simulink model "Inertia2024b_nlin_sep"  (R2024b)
settings: Solver=ode1  StartTime=0.0  StopTime=30  FixedStep=Tstep  EnableMultiTasking=on
model workspace (MAT data in the model file):
  op_snapshot1 : opcond.OperatingPoint (value not decoded)
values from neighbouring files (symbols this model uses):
  T_dis = 2.5    [onebus_nonlinsub.m]
  Ts = Tstep    (= 1e-05)    [onebus_nonlinsub.m]    (also in DemoMTI_Boolean_Index_MTI.m = 1; DemoMTI_EKF.m = 0.02; DemoMTI_MHE_VanDePol.m = 0.01)
  Tstep = 1e-5    (= 1e-05)    [DemoMTI_greyestGFM.m]    (also in onebus_nonlinsub.m)
  Vn = 380    [simulink_parameters_one_bus.m]    (also in nine_bus_parameters.m = 310.*ones(num_inv,1))
  Vtri = Vdc1./3    [simulink_parameters_one_bus.m]    (also in nine_bus_parameters.m = Vdc./2)
  wn = ones(num_inv,1).*w01    [nine_bus_parameters.m]    (also in computeModeFrequencyDampingTable.m = abs(lambda))
undefined symbols (not defined in the file or in its folder): D1_g1, Dsg, Dxd, Dxq, Efdmax_g1, Efdmin_g1, Ibg, K_int_pll, K_prop_pll, KA_g1, kpss_g1, L_1_2, M1_g1, Msg, nom, op, R_1_2, ra_g1, Rsg, T1_g1, T2_g1, T3_g1, T4_g1, TA_g1, Td, Td0p_g1, Tq0p_g1, Tv, Tw_g1, Vbg, xdp_g1, xqp_g1
libraries: spsThreePhaseVIMeasurementLib x5, spsGroundLib x4, slpidlib x4, spsControlledVoltageSourceLib x3, spsControlledCurrentSourceLib x3, spsSeriesRLCBranchLib x3, spsThreePhaseSeriesRLCBranchLib x2, spsThreePhaseSeriesRLCLoadLib x2, spsThreePhaseTransformerTwoWindingsLib x1, spsThreePhaseDynamicLoadLib x1, spsSampleandHoldLib x1, sps_lib x1
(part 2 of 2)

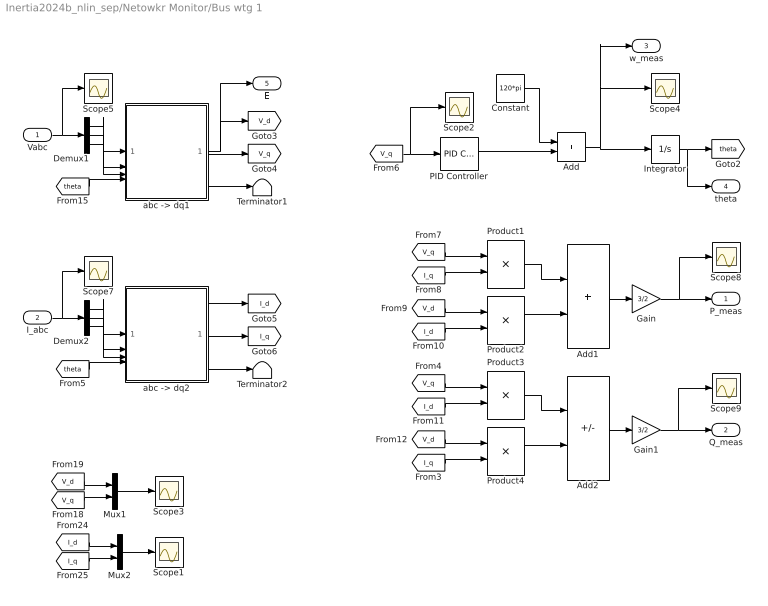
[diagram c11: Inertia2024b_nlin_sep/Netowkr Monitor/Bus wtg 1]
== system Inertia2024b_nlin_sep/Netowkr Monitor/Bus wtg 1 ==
  Vabc : Inport
  I_abc : Inport  Port=2
  Add : Sum
  Add1 : Sum
  Add2 : Sum  Inputs=+-
  Constant : Constant  Value=120*pi
  Demux1 : Demux  Outputs=3
  Demux2 : Demux  Outputs=3
  Gain : Gain  Gain=3/2
  Gain1 : Gain  Gain=3/2
  Integrator : Integrator  IgnoreLimit=on
  Mux1 : Mux  Inputs=2
  Mux2 : Mux  Inputs=2
  PID Controller : slpidlib/PID Controller  Controller=PI  Form=Parallel  TimeDomain=Continuous-time  UseExternalTs=off  SampleTime=-1  IntegratorMethod=Forward Euler  FilterMethod=Forward Euler  ControllerParametersSource=internal  P=K_prop_pll  I=K_int_pll  UseKiTs=off  D=0  UseExternalDerivativeSource=off  N=100  UseFilter=on  TunerSelectOption=Transfer Function Based (PID Tuner App)  InitialConditionSource=internal  InitialConditionForIntegrator=0  InitialConditionForFilter=0  DifferentiatorICPrevScaledInput=0  ExternalReset=none  IgnoreLimit=on  TrackingMode=off  Kt=1  LimitOutput=off  SatLimitsSource=internal  UpperSaturationLimit=inf  LowerSaturationLimit=-inf  LinearizeAsGain=on  AntiWindupMode=none  Kb=1  LimitIntegrator=off  UpperIntegratorSaturationLimit=inf  LowerIntegratorSaturationLimit=-inf  POutMin=[]  POutMax=[]  IOutMin=[]  IOutMax=[]  DOutMin=[]  DOutMax=[]  NOutMin=[]  NOutMax=[]  SumOutMin=[]  SumOutMax=[]  SaturationOutMin=[]  SaturationOutMax=[]  PParamMin=[]  PParamMax=[]  IParamMin=[]  IParamMax=[]  DParamMin=[]  DParamMax=[]  NParamMin=[]  NParamMax=[]  KbParamMin=[]  KbParamMax=[]  KtParamMin=[]  KtParamMax=[]  KbOutMin=[]  KbOutMax=[]  KtOutMin=[]  KtOutMax=[]  IntegratorOutMin=[]  IntegratorOutMax=[]  FilterOutMin=[]  FilterOutMax=[]  SumI1OutMin=[]  SumI1OutMax=[]  SumI2OutMin=[]  SumI2OutMax=[]  SumI3OutMin=[]  SumI3OutMax=[]  SumI4OutMin=[]  SumI4OutMax=[]  SumDOutMin=[]  SumDOutMax=[]  DifferentiatorOutMin=[]  DifferentiatorOutMax=[]  FilterDiffOutCoefMin=[]  FilterDiffOutCoefMax=[]  ReciprocalOutMin=[]  ReciprocalOutMax=[]  SumDenOutMin=[]  SumDenOutMax=[]  SumNumOutMin=[]  SumNumOutMax=[]  DivideOutMin=[]  DivideOutMax=[]  UdiffTsProdOutMin=[]  UdiffTsProdOutMax=[]  NTsProdOutMin=[]  NTsProdOutMax=[]  UintegralTsProdOutMin=[]  UintegralTsProdOutMax=[]  UngainTsProdOutMin=[]  UngainTsProdOutMax=[]  ClampingZeroOutDataTypeStr=Inherit: Inherit via back propagation  ClampingZeroOutMin=[]  ClampingZeroOutMax=[]  FilterDenConstantOutDataTypeStr=Inherit: Inherit via back propagation  FilterDenConstantOutMin=[]  FilterDenConstantOutMax=[]  PCopyOutDataTypeStr=Inherit: Inherit via back propagation  PCopyOutMin=[]  PCopyOutMax=[]  NCopyOutDataTypeStr=Inherit: Inherit via back propagation  NCopyOutMin=[]  NCopyOutMax=[]  IntegratorContinuousStateAttributes=''  IntegratorStateMustResolveToSignalObject=off  IntegratorRTWStateStorageClass=Auto  FilterContinuousStateAttributes=''  FilterStateMustResolveToSignalObject=off  FilterRTWStateStorageClass=Auto  ParallelPVariant=InternalParameters  IdealPVariant=Disabled  IVariant=InternalParameters  DVariant=Disabled  IntegratorVariant=Continuous  SatVariant=Disabled  AWVariant=Passthrough  PCopyVariant=Disabled  TRVariant=Disabled  FdbkBlocksVariant=Forward  IdealPFdbkVariant=Disabled  SatFdbkVariant=Disabled  DerivativeFilterVariant=Disabled  NVariant=Disabled  NCopyVariant=Disabled_SignalSpec  FilterICVariant=Disabled  IntegratorICVariant=InternalICs  ExternalResetVariant=Disabled  TRSumVariant=Passthrough  SumFdbkVariant=Disabled  SumVariant=Sum_PI  TsampFilterVariant=InternalTs  TsampNgainVariant=Passthrough  TsampIntegralVariant=Disabled_SignalSpec  ExternalSaturationOutDataTypeStr=Inherit: Same as second input  DerivativeSourceVariant=Disabled  PreIntVariant=InternalPreInt
  Product{1..4} (4 alike) : Product
  Scope{1..5,7..9} (8 alike) : Scope
  Terminator1 : Terminator
  Terminator2 : Terminator
  "abc -> dq1" : Subsystem
  "abc -> dq2" : Subsystem
  P_meas : Outport  VectorParamsAs1DForOutWhenUnconnected=off
  Q_meas : Outport  Port=2  VectorParamsAs1DForOutWhenUnconnected=off
  w_meas : Outport  Port=3  VectorParamsAs1DForOutWhenUnconnected=off
  theta : Outport  Port=4  VectorParamsAs1DForOutWhenUnconnected=off
  E : Outport  Port=5  VectorParamsAs1DForOutWhenUnconnected=off
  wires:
  Add/1 -> Integrator/1, w_meas/1, Scope4/1
  [V_q] -> Scope2/1, PID Controller/1
  PID Controller/1 -> Add/2
  Constant/1 -> Add/1
  Demux1/2 -> "abc -> dq1"/2(b)
  Demux1/3 -> "abc -> dq1"/3(c)
  [theta] -> "abc -> dq1"/4(Theta)
  Vabc/1 -> Scope5/1, Demux1/1
  Demux1/1 -> "abc -> dq1"/1(a)
  "abc -> dq1"/3(0) -> Terminator1/1
  "abc -> dq1"/2(q) -> [V_q]
  Integrator/1 -> theta/1, [theta]
  Demux2/2 -> "abc -> dq2"/2(b)
  Demux2/3 -> "abc -> dq2"/3(c)
  [theta] -> "abc -> dq2"/4(Theta)
  I_abc/1 -> Scope7/1, Demux2/1
  Demux2/1 -> "abc -> dq2"/1(a)
  "abc -> dq2"/3(0) -> Terminator2/1
  "abc -> dq2"/2(q) -> [I_q]
  "abc -> dq2"/1(d) -> [I_d]
  [V_q] -> Product1/1
  [I_q] -> Product1/2
  Product1/1 -> Add1/1
  [V_d] -> Product2/1
  [I_d] -> Product2/2
  Product2/1 -> Add1/2
  Add1/1 -> Gain/1
  Gain/1 -> Scope8/1, P_meas/1
  [V_q] -> Product3/1
  [I_d] -> Product3/2
  Product3/1 -> Add2/1
  [V_d] -> Product4/1
  [I_q] -> Product4/2
  Product4/1 -> Add2/2
  Add2/1 -> Gain1/1
  Gain1/1 -> Scope9/1, Q_meas/1
  [V_d] -> Mux1/1
  [I_d] -> Mux2/1
  [I_q] -> Mux2/2
  [V_q] -> Mux1/2
  Mux1/1 -> Scope3/1
  Mux2/1 -> Scope1/1
  "abc -> dq1"/1(d) -> E/1, [V_d]

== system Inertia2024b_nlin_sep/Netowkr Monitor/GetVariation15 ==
  In1 : Inport
  Minus : Sum  Inputs=|+-
  Sample and Hold2 : spsSampleandHoldLib/Sample and Hold  ic=0  Ts=Ts
  Scope17 : Scope
  Out1 : Outport  VectorParamsAs1DForOutWhenUnconnected=off
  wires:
  Sample and Hold2/1 -> Scope17/1, Minus/2
  [op_hold] -> Sample and Hold2/2
  In1/1 -> Sample and Hold2/1, Minus/1
  Minus/1 -> Out1/1

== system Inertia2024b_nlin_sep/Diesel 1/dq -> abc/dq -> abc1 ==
  d : Inport
  q : Inport  Port=2
  Theta : Inport  Port=3
  Add1 : Sum  Inputs=+++
  Add10 : Sum  Inputs=+++
  Add11 : Sum  Inputs=+++
  Add4 : Sum  Inputs=+-
  Add8 : Sum
  Constant6 : Constant  Value=2/3*pi
  Constant7 : Constant  Value=2/3*pi
  Divide{6..11} (6 alike) : Product  Inputs=**
  Trigonometric Function : Trigonometry  Operator=cos
  Trigonometric Function1 : Trigonometry  Operator=cos
  Trigonometric Function2 : Trigonometry  Operator=cos
  Trigonometric Function3 : Trigonometry
  Trigonometric Function4 : Trigonometry
  Trigonometric Function5 : Trigonometry
  a : Outport  VectorParamsAs1DForOutWhenUnconnected=off
  b : Outport  Port=2  VectorParamsAs1DForOutWhenUnconnected=off
  c : Outport  Port=3  VectorParamsAs1DForOutWhenUnconnected=off
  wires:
  Add11/1 -> b/1
  Add10/1 -> a/1
  Divide9/1 -> Add11/2
  Divide6/1 -> Add10/1
  Constant7/1 -> Add8/2
  Trigonometric Function1/1 -> Divide8/2
  Trigonometric Function2/1 -> Divide10/2
  Trigonometric Function/1 -> Divide6/2
  Trigonometric Function5/1 -> Divide11/2
  Trigonometric Function4/1 -> Divide9/2
  Trigonometric Function3/1 -> Divide7/2
  Add8/1 -> Trigonometric Function5/1, Trigonometric Function2/1
  Add4/1 -> Trigonometric Function4/1, Trigonometric Function1/1
  Constant6/1 -> Add4/2
  Theta/1 -> Trigonometric Function3/1, Trigonometric Function/1, Add8/1, Add4/1  "wt"
  q/1 -> Divide6/1, Divide8/1, Divide10/1
  Add1/1 -> c/1
  Divide7/1 -> Add10/2
  d/1 -> Divide7/1, Divide9/1, Divide11/1
  Divide8/1 -> Add11/1
  Divide11/1 -> Add1/2
  Divide10/1 -> Add1/1

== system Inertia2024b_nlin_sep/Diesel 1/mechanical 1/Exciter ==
  Vt : Inport
  Vtr0 : Inport  Port=2
  Vpss : Inport  Port=3
  Add : Sum  Inputs=++-
  Mux4 : Mux  Commented=on  Inputs=2
  Saturation : Saturate  UpperLimit=Efdmax_g1  LowerLimit=Efdmin_g1
  Scope1 : Scope
  Scope2 : Scope
  Scope3 : Scope
  State-Space1 : StateSpace  A=-1/TA_g1  B=KA_g1/TA_g1  D=0  InitialCondition=0
  Transfer Fcn : TransferFcn  Commented=on  Numerator=[KA_g1]  Denominator="[TA_g1  1]"
  Ef : Outport  VectorParamsAs1DForOutWhenUnconnected=off
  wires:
  Vpss/1 -> Add/2
  Vt/1 -> Add/3
  Vtr0/1 -> Add/1
  Saturation/1 -> Ef/1
  State-Space1/1 -> Mux4/1, Scope3/1, Saturation/1
  Add/1 -> Scope1/1, Transfer Fcn/1, State-Space1/1
  Mux4/1 -> Scope2/1
  Transfer Fcn/1 -> Mux4/2

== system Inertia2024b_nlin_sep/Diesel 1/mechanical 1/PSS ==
  dw : Inport
  Gain : Gain  Gain=kpss_g1
  Mux : Mux  Commented=on  Inputs=2
  Mux1 : Mux  Commented=on  Inputs=2
  Mux2 : Mux  Commented=on  Inputs=2
  Scope : Scope
  Scope1 : Scope
  Scope2 : Scope
  State-Space : StateSpace  A=-1/Tw_g1  B=1/Tw_g1  C=-1  InitialCondition=0
  State-Space1 : StateSpace  A=-1/T2_g1  B=T1_g1/T2_g1-1  C=-1/T2_g1  D=T1_g1/T2_g1  InitialCondition=0
  State-Space2 : StateSpace  A=-1/T4_g1  B=T3_g1/T4_g1-1  C=-1/T4_g1  D=T3_g1/T4_g1  InitialCondition=0
  Transfer Fcn : TransferFcn  Commented=on  Numerator=[Tw_g1 0]  Denominator=[Tw_g1 1]
  Transfer Fcn1 : TransferFcn  Commented=on  Numerator=[T1_g1 1]  Denominator=[T2_g1 1]
  Transfer Fcn2 : TransferFcn  Commented=on  Numerator=[T3_g1 1]  Denominator=[T4_g1 1]
  Vpss : Outport  VectorParamsAs1DForOutWhenUnconnected=off
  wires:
  dw/1 -> Gain/1
  Gain/1 -> Transfer Fcn/1, State-Space/1
  State-Space/1 -> Mux/1, State-Space1/1
  Transfer Fcn/1 -> Mux/2, Transfer Fcn1/1
  Mux/1 -> Scope/1
  State-Space1/1 -> Mux1/1, State-Space2/1
  Transfer Fcn1/1 -> Mux1/2, Transfer Fcn2/1
  Mux1/1 -> Scope1/1
  State-Space2/1 -> Mux2/1, Vpss/1
  Transfer Fcn2/1 -> Mux2/2
  Mux2/1 -> Scope2/1

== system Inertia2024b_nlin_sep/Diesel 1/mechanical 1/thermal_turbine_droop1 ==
  dw : Inport
  pe : Inport  Port=2
  Constant1 : Constant  Value=0
  Engine : StateSpace  A=-1/Td(1)  B=1/Td(1)  D=0  InitialCondition=op.Pm
  Mux : Mux  Inputs=2
  Mux2 : Mux  Commented=on  Inputs=2
  Mux3 : Mux  Commented=on  Inputs=2
  Mux4 : Mux  Commented=on  Inputs=2
  Saturation : Saturate  UpperLimit=10  LowerLimit=-10
  Saturation1 : Saturate  UpperLimit=10  LowerLimit=-10
  Scope{,1..5} (6 alike) : Scope
  Sum : Sum  Inputs=+-|
  Sum1 : Sum  Inputs=-+|
  Sum2 : Sum  Inputs=-+|
  Swing : StateSpace  A=(-Dsg(1)*60)/Msg(1)  B=(1*60)/Msg(1)  D=0  InitialCondition=0
  Swing1 : StateSpace  A=(-Dsg(1))/Msg(1)  B=(1)/Msg(1)  D=0  InitialCondition=0
  Transfer Fcn : TransferFcn  Commented=on  Denominator=[Tv 1]
  Transfer Fcn1 : TransferFcn  Commented=on  Denominator=[Td 1]
  Transfer Fcn2 : TransferFcn  Commented=on  Denominator=[M1_g1 D1_g1]
  Vale : StateSpace  A=-1/Tv(1)  B=1/Tv(1)  D=0  InitialCondition=op.Pc
  droop : Gain  Gain=Rsg(1)*(1/60)
  dww : Outport  VectorParamsAs1DForOutWhenUnconnected=off
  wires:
  Vale/1 -> Scope5/1, Saturation/1
  Sum/1 -> Vale/1
  dw/1 -> droop/1
  Engine/1 -> Scope3/1, Saturation1/1  "Pm"
  droop/1 -> Sum/2
  Transfer Fcn/1 -> Mux4/2, Transfer Fcn1/1
  Mux3/1 -> Scope/1
  Transfer Fcn2/1 -> Mux3/2
  Mux2/1 -> Scope1/1
  Transfer Fcn1/1 -> Mux2/2
  Mux4/1 -> Scope2/1
  pe/1 -> Sum1/1  "Pe"
  Sum1/1 -> Swing/1
  Constant1/1 -> Sum/1
  Saturation/1 -> Engine/1, [Pv1]
  Saturation1/1 -> Mux/2, [Pm1], Sum1/2  "Pm"
  Swing/1 -> dww/1
  Mux/1 -> Scope4/1

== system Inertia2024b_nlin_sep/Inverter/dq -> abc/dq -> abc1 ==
  d : Inport
  q : Inport  Port=2
  Theta : Inport  Port=3
  Add1 : Sum  Inputs=+++
  Add10 : Sum  Inputs=+++
  Add11 : Sum  Inputs=+++
  Add4 : Sum  Inputs=+-
  Add8 : Sum
  Constant6 : Constant  Value=2/3*pi
  Constant7 : Constant  Value=2/3*pi
  Divide{6..11} (6 alike) : Product  Inputs=**
  Trigonometric Function : Trigonometry  Operator=cos
  Trigonometric Function1 : Trigonometry  Operator=cos
  Trigonometric Function2 : Trigonometry  Operator=cos
  Trigonometric Function3 : Trigonometry
  Trigonometric Function4 : Trigonometry
  Trigonometric Function5 : Trigonometry
  a : Outport  VectorParamsAs1DForOutWhenUnconnected=off
  b : Outport  Port=2  VectorParamsAs1DForOutWhenUnconnected=off
  c : Outport  Port=3  VectorParamsAs1DForOutWhenUnconnected=off
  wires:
  Add11/1 -> b/1
  Add10/1 -> a/1
  Divide9/1 -> Add11/2
  Divide6/1 -> Add10/1
  Constant7/1 -> Add8/2
  Trigonometric Function1/1 -> Divide8/2
  Trigonometric Function2/1 -> Divide10/2
  Trigonometric Function/1 -> Divide6/2
  Trigonometric Function5/1 -> Divide11/2
  Trigonometric Function4/1 -> Divide9/2
  Trigonometric Function3/1 -> Divide7/2
  Add8/1 -> Trigonometric Function5/1, Trigonometric Function2/1
  Add4/1 -> Trigonometric Function4/1, Trigonometric Function1/1
  Constant6/1 -> Add4/2
  Theta/1 -> Trigonometric Function3/1, Trigonometric Function/1, Add8/1, Add4/1  "wt"
  q/1 -> Divide6/1, Divide8/1, Divide10/1
  Add1/1 -> c/1
  Divide7/1 -> Add10/2
  d/1 -> Divide7/1, Divide9/1, Divide11/1
  Divide8/1 -> Add11/1
  Divide11/1 -> Add1/2
  Divide10/1 -> Add1/1

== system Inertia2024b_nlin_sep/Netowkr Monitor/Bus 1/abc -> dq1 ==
  a : Inport
  b : Inport  Port=2
  c : Inport  Port=3
  Theta : Inport  Port=4
  Add1 : Sum  Inputs=+++
  Add10 : Sum  Inputs=+++
  Add11 : Sum  Inputs=+++
  Add4 : Sum  Inputs=+-
  Add8 : Sum
  Constant6 : Constant  Value=2/3*pi
  Constant7 : Constant  Value=2/3*pi
  Divide{6..11} (6 alike) : Product  Inputs=**
  Gain6 : Gain  Gain=1/3
  Mux1 : Mux  Inputs=2
  Scope3 : Scope
  Trigonometric Function : Trigonometry  Operator=cos
  Trigonometric Function1 : Trigonometry  Operator=cos
  Trigonometric Function2 : Trigonometry  Operator=cos
  Trigonometric Function3 : Trigonometry
  Trigonometric Function4 : Trigonometry
  Trigonometric Function5 : Trigonometry
  Vd : Gain  Gain=2/3
  Vq : Gain  Gain=2/3
  d : Outport  VectorParamsAs1DForOutWhenUnconnected=off
  q : Outport  Port=2  VectorParamsAs1DForOutWhenUnconnected=off
  0 : Outport  Port=3  VectorParamsAs1DForOutWhenUnconnected=off
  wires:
  Theta/1 -> Add4/1, Add8/1, Trigonometric Function/1, Trigonometric Function3/1  "wt"
  Constant6/1 -> Add4/2
  Add4/1 -> Trigonometric Function1/1, Trigonometric Function4/1
  Add8/1 -> Trigonometric Function2/1, Trigonometric Function5/1
  Trigonometric Function3/1 -> Divide7/2
  Trigonometric Function4/1 -> Divide9/2
  Trigonometric Function5/1 -> Divide11/2
  a/1 -> Divide6/1, Divide7/1, Add1/1
  Trigonometric Function/1 -> Divide6/2
  Trigonometric Function2/1 -> Divide10/2
  Trigonometric Function1/1 -> Divide8/2
  b/1 -> Divide8/1, Divide9/1, Add1/2
  c/1 -> Divide10/1, Divide11/1, Add1/3
  Constant7/1 -> Add8/2
  Divide6/1 -> Add10/1
  Divide8/1 -> Add10/2
  Divide10/1 -> Add10/3
  Divide7/1 -> Add11/1
  Divide9/1 -> Add11/2
  Divide11/1 -> Add11/3
  Add10/1 -> Vq/1
  Add11/1 -> Vd/1
  Vq/1 -> Mux1/2, q/1
  Vd/1 -> Mux1/1, d/1
  Add1/1 -> Gain6/1
  Gain6/1 -> 0/1
  Mux1/1 -> Scope3/1

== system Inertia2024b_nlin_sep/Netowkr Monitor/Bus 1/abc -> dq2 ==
  a : Inport
  b : Inport  Port=2
  c : Inport  Port=3
  Theta : Inport  Port=4
  Add1 : Sum  Inputs=+++
  Add10 : Sum  Inputs=+++
  Add11 : Sum  Inputs=+++
  Add4 : Sum  Inputs=+-
  Add8 : Sum
  Constant6 : Constant  Value=2/3*pi
  Constant7 : Constant  Value=2/3*pi
  Divide{6..11} (6 alike) : Product  Inputs=**
  Gain6 : Gain  Gain=1/3
  Mux1 : Mux  Inputs=2
  Scope3 : Scope
  Trigonometric Function : Trigonometry  Operator=cos
  Trigonometric Function1 : Trigonometry  Operator=cos
  Trigonometric Function2 : Trigonometry  Operator=cos
  Trigonometric Function3 : Trigonometry
  Trigonometric Function4 : Trigonometry
  Trigonometric Function5 : Trigonometry
  Vd : Gain  Gain=2/3
  Vq : Gain  Gain=2/3
  d : Outport  VectorParamsAs1DForOutWhenUnconnected=off
  q : Outport  Port=2  VectorParamsAs1DForOutWhenUnconnected=off
  0 : Outport  Port=3  VectorParamsAs1DForOutWhenUnconnected=off
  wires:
  Theta/1 -> Add4/1, Add8/1, Trigonometric Function/1, Trigonometric Function3/1  "wt"
  Constant6/1 -> Add4/2
  Add4/1 -> Trigonometric Function1/1, Trigonometric Function4/1
  Add8/1 -> Trigonometric Function2/1, Trigonometric Function5/1
  Trigonometric Function3/1 -> Divide7/2
  Trigonometric Function4/1 -> Divide9/2
  Trigonometric Function5/1 -> Divide11/2
  a/1 -> Divide6/1, Divide7/1, Add1/1
  Trigonometric Function/1 -> Divide6/2
  Trigonometric Function2/1 -> Divide10/2
  Trigonometric Function1/1 -> Divide8/2
  b/1 -> Divide8/1, Divide9/1, Add1/2
  c/1 -> Divide10/1, Divide11/1, Add1/3
  Constant7/1 -> Add8/2
  Divide6/1 -> Add10/1
  Divide8/1 -> Add10/2
  Divide10/1 -> Add10/3
  Divide7/1 -> Add11/1
  Divide9/1 -> Add11/2
  Divide11/1 -> Add11/3
  Add10/1 -> Vq/1
  Add11/1 -> Vd/1
  Vq/1 -> Mux1/2, q/1
  Vd/1 -> Mux1/1, d/1
  Add1/1 -> Gain6/1
  Gain6/1 -> 0/1
  Mux1/1 -> Scope3/1

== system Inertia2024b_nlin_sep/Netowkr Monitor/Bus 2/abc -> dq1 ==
  a : Inport
  b : Inport  Port=2
  c : Inport  Port=3
  Theta : Inport  Port=4
  Add1 : Sum  Inputs=+++
  Add10 : Sum  Inputs=+++
  Add11 : Sum  Inputs=+++
  Add4 : Sum  Inputs=+-
  Add8 : Sum
  Constant6 : Constant  Value=2/3*pi
  Constant7 : Constant  Value=2/3*pi
  Divide{6..11} (6 alike) : Product  Inputs=**
  Gain6 : Gain  Gain=1/3
  Mux1 : Mux  Inputs=2
  Scope3 : Scope
  Trigonometric Function : Trigonometry  Operator=cos
  Trigonometric Function1 : Trigonometry  Operator=cos
  Trigonometric Function2 : Trigonometry  Operator=cos
  Trigonometric Function3 : Trigonometry
  Trigonometric Function4 : Trigonometry
  Trigonometric Function5 : Trigonometry
  Vd : Gain  Gain=2/3
  Vq : Gain  Gain=2/3
  d : Outport  VectorParamsAs1DForOutWhenUnconnected=off
  q : Outport  Port=2  VectorParamsAs1DForOutWhenUnconnected=off
  0 : Outport  Port=3  VectorParamsAs1DForOutWhenUnconnected=off
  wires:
  Theta/1 -> Add4/1, Add8/1, Trigonometric Function/1, Trigonometric Function3/1  "wt"
  Constant6/1 -> Add4/2
  Add4/1 -> Trigonometric Function1/1, Trigonometric Function4/1
  Add8/1 -> Trigonometric Function2/1, Trigonometric Function5/1
  Trigonometric Function3/1 -> Divide7/2
  Trigonometric Function4/1 -> Divide9/2
  Trigonometric Function5/1 -> Divide11/2
  a/1 -> Divide6/1, Divide7/1, Add1/1
  Trigonometric Function/1 -> Divide6/2
  Trigonometric Function2/1 -> Divide10/2
  Trigonometric Function1/1 -> Divide8/2
  b/1 -> Divide8/1, Divide9/1, Add1/2
  c/1 -> Divide10/1, Divide11/1, Add1/3
  Constant7/1 -> Add8/2
  Divide6/1 -> Add10/1
  Divide8/1 -> Add10/2
  Divide10/1 -> Add10/3
  Divide7/1 -> Add11/1
  Divide9/1 -> Add11/2
  Divide11/1 -> Add11/3
  Add10/1 -> Vq/1
  Add11/1 -> Vd/1
  Vq/1 -> Mux1/2, q/1
  Vd/1 -> Mux1/1, d/1
  Add1/1 -> Gain6/1
  Gain6/1 -> 0/1
  Mux1/1 -> Scope3/1

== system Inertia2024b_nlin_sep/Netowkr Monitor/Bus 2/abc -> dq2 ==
  a : Inport
  b : Inport  Port=2
  c : Inport  Port=3
  Theta : Inport  Port=4
  Add1 : Sum  Inputs=+++
  Add10 : Sum  Inputs=+++
  Add11 : Sum  Inputs=+++
  Add4 : Sum  Inputs=+-
  Add8 : Sum
  Constant6 : Constant  Value=2/3*pi
  Constant7 : Constant  Value=2/3*pi
  Divide{6..11} (6 alike) : Product  Inputs=**
  Gain6 : Gain  Gain=1/3
  Mux1 : Mux  Inputs=2
  Scope3 : Scope
  Trigonometric Function : Trigonometry  Operator=cos
  Trigonometric Function1 : Trigonometry  Operator=cos
  Trigonometric Function2 : Trigonometry  Operator=cos
  Trigonometric Function3 : Trigonometry
  Trigonometric Function4 : Trigonometry
  Trigonometric Function5 : Trigonometry
  Vd : Gain  Gain=2/3
  Vq : Gain  Gain=2/3
  d : Outport  VectorParamsAs1DForOutWhenUnconnected=off
  q : Outport  Port=2  VectorParamsAs1DForOutWhenUnconnected=off
  0 : Outport  Port=3  VectorParamsAs1DForOutWhenUnconnected=off
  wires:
  Theta/1 -> Add4/1, Add8/1, Trigonometric Function/1, Trigonometric Function3/1  "wt"
  Constant6/1 -> Add4/2
  Add4/1 -> Trigonometric Function1/1, Trigonometric Function4/1
  Add8/1 -> Trigonometric Function2/1, Trigonometric Function5/1
  Trigonometric Function3/1 -> Divide7/2
  Trigonometric Function4/1 -> Divide9/2
  Trigonometric Function5/1 -> Divide11/2
  a/1 -> Divide6/1, Divide7/1, Add1/1
  Trigonometric Function/1 -> Divide6/2
  Trigonometric Function2/1 -> Divide10/2
  Trigonometric Function1/1 -> Divide8/2
  b/1 -> Divide8/1, Divide9/1, Add1/2
  c/1 -> Divide10/1, Divide11/1, Add1/3
  Constant7/1 -> Add8/2
  Divide6/1 -> Add10/1
  Divide8/1 -> Add10/2
  Divide10/1 -> Add10/3
  Divide7/1 -> Add11/1
  Divide9/1 -> Add11/2
  Divide11/1 -> Add11/3
  Add10/1 -> Vq/1
  Add11/1 -> Vd/1
  Vq/1 -> Mux1/2, q/1
  Vd/1 -> Mux1/1, d/1
  Add1/1 -> Gain6/1
  Gain6/1 -> 0/1
  Mux1/1 -> Scope3/1

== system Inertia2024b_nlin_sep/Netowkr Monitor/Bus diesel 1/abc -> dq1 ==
  a : Inport
  b : Inport  Port=2
  c : Inport  Port=3
  Theta : Inport  Port=4
  Add1 : Sum  Inputs=+++
  Add10 : Sum  Inputs=+++
  Add11 : Sum  Inputs=+++
  Add4 : Sum  Inputs=+-
  Add8 : Sum
  Constant6 : Constant  Value=2/3*pi
  Constant7 : Constant  Value=2/3*pi
  Divide{6..11} (6 alike) : Product  Inputs=**
  Gain6 : Gain  Gain=1/3
  Mux1 : Mux  Inputs=2
  Scope3 : Scope
  Trigonometric Function : Trigonometry  Operator=cos
  Trigonometric Function1 : Trigonometry  Operator=cos
  Trigonometric Function2 : Trigonometry  Operator=cos
  Trigonometric Function3 : Trigonometry
  Trigonometric Function4 : Trigonometry
  Trigonometric Function5 : Trigonometry
  Vd : Gain  Gain=2/3
  Vq : Gain  Gain=2/3
  d : Outport  VectorParamsAs1DForOutWhenUnconnected=off
  q : Outport  Port=2  VectorParamsAs1DForOutWhenUnconnected=off
  0 : Outport  Port=3  VectorParamsAs1DForOutWhenUnconnected=off
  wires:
  Theta/1 -> Add4/1, Add8/1, Trigonometric Function/1, Trigonometric Function3/1  "wt"
  Constant6/1 -> Add4/2
  Add4/1 -> Trigonometric Function1/1, Trigonometric Function4/1
  Add8/1 -> Trigonometric Function2/1, Trigonometric Function5/1
  Trigonometric Function3/1 -> Divide7/2
  Trigonometric Function4/1 -> Divide9/2
  Trigonometric Function5/1 -> Divide11/2
  a/1 -> Divide6/1, Divide7/1, Add1/1
  Trigonometric Function/1 -> Divide6/2
  Trigonometric Function2/1 -> Divide10/2
  Trigonometric Function1/1 -> Divide8/2
  b/1 -> Divide8/1, Divide9/1, Add1/2
  c/1 -> Divide10/1, Divide11/1, Add1/3
  Constant7/1 -> Add8/2
  Divide6/1 -> Add10/1
  Divide8/1 -> Add10/2
  Divide10/1 -> Add10/3
  Divide7/1 -> Add11/1
  Divide9/1 -> Add11/2
  Divide11/1 -> Add11/3
  Add10/1 -> Vq/1
  Add11/1 -> Vd/1
  Vq/1 -> Mux1/2, q/1
  Vd/1 -> Mux1/1, d/1
  Add1/1 -> Gain6/1
  Gain6/1 -> 0/1
  Mux1/1 -> Scope3/1

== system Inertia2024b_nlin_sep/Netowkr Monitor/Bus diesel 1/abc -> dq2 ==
  a : Inport
  b : Inport  Port=2
  c : Inport  Port=3
  Theta : Inport  Port=4
  Add1 : Sum  Inputs=+++
  Add10 : Sum  Inputs=+++
  Add11 : Sum  Inputs=+++
  Add4 : Sum  Inputs=+-
  Add8 : Sum
  Constant6 : Constant  Value=2/3*pi
  Constant7 : Constant  Value=2/3*pi
  Divide{6..11} (6 alike) : Product  Inputs=**
  Gain6 : Gain  Gain=1/3
  Mux1 : Mux  Inputs=2
  Scope3 : Scope
  Trigonometric Function : Trigonometry  Operator=cos
  Trigonometric Function1 : Trigonometry  Operator=cos
  Trigonometric Function2 : Trigonometry  Operator=cos
  Trigonometric Function3 : Trigonometry
  Trigonometric Function4 : Trigonometry
  Trigonometric Function5 : Trigonometry
  Vd : Gain  Gain=2/3
  Vq : Gain  Gain=2/3
  d : Outport  VectorParamsAs1DForOutWhenUnconnected=off
  q : Outport  Port=2  VectorParamsAs1DForOutWhenUnconnected=off
  0 : Outport  Port=3  VectorParamsAs1DForOutWhenUnconnected=off
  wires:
  Theta/1 -> Add4/1, Add8/1, Trigonometric Function/1, Trigonometric Function3/1  "wt"
  Constant6/1 -> Add4/2
  Add4/1 -> Trigonometric Function1/1, Trigonometric Function4/1
  Add8/1 -> Trigonometric Function2/1, Trigonometric Function5/1
  Trigonometric Function3/1 -> Divide7/2
  Trigonometric Function4/1 -> Divide9/2
  Trigonometric Function5/1 -> Divide11/2
  a/1 -> Divide6/1, Divide7/1, Add1/1
  Trigonometric Function/1 -> Divide6/2
  Trigonometric Function2/1 -> Divide10/2
  Trigonometric Function1/1 -> Divide8/2
  b/1 -> Divide8/1, Divide9/1, Add1/2
  c/1 -> Divide10/1, Divide11/1, Add1/3
  Constant7/1 -> Add8/2
  Divide6/1 -> Add10/1
  Divide8/1 -> Add10/2
  Divide10/1 -> Add10/3
  Divide7/1 -> Add11/1
  Divide9/1 -> Add11/2
  Divide11/1 -> Add11/3
  Add10/1 -> Vq/1
  Add11/1 -> Vd/1
  Vq/1 -> Mux1/2, q/1
  Vd/1 -> Mux1/1, d/1
  Add1/1 -> Gain6/1
  Gain6/1 -> 0/1
  Mux1/1 -> Scope3/1

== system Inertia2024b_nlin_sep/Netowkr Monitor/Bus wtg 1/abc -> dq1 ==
  a : Inport
  b : Inport  Port=2
  c : Inport  Port=3
  Theta : Inport  Port=4
  Add1 : Sum  Inputs=+++
  Add10 : Sum  Inputs=+++
  Add11 : Sum  Inputs=+++
  Add4 : Sum  Inputs=+-
  Add8 : Sum
  Constant6 : Constant  Value=2/3*pi
  Constant7 : Constant  Value=2/3*pi
  Divide{6..11} (6 alike) : Product  Inputs=**
  Gain6 : Gain  Gain=1/3
  Mux1 : Mux  Inputs=2
  Scope3 : Scope
  Trigonometric Function : Trigonometry  Operator=cos
  Trigonometric Function1 : Trigonometry  Operator=cos
  Trigonometric Function2 : Trigonometry  Operator=cos
  Trigonometric Function3 : Trigonometry
  Trigonometric Function4 : Trigonometry
  Trigonometric Function5 : Trigonometry
  Vd : Gain  Gain=2/3
  Vq : Gain  Gain=2/3
  d : Outport  VectorParamsAs1DForOutWhenUnconnected=off
  q : Outport  Port=2  VectorParamsAs1DForOutWhenUnconnected=off
  0 : Outport  Port=3  VectorParamsAs1DForOutWhenUnconnected=off
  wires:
  Theta/1 -> Add4/1, Add8/1, Trigonometric Function/1, Trigonometric Function3/1  "wt"
  Constant6/1 -> Add4/2
  Add4/1 -> Trigonometric Function1/1, Trigonometric Function4/1
  Add8/1 -> Trigonometric Function2/1, Trigonometric Function5/1
  Trigonometric Function3/1 -> Divide7/2
  Trigonometric Function4/1 -> Divide9/2
  Trigonometric Function5/1 -> Divide11/2
  a/1 -> Divide6/1, Divide7/1, Add1/1
  Trigonometric Function/1 -> Divide6/2
  Trigonometric Function2/1 -> Divide10/2
  Trigonometric Function1/1 -> Divide8/2
  b/1 -> Divide8/1, Divide9/1, Add1/2
  c/1 -> Divide10/1, Divide11/1, Add1/3
  Constant7/1 -> Add8/2
  Divide6/1 -> Add10/1
  Divide8/1 -> Add10/2
  Divide10/1 -> Add10/3
  Divide7/1 -> Add11/1
  Divide9/1 -> Add11/2
  Divide11/1 -> Add11/3
  Add10/1 -> Vq/1
  Add11/1 -> Vd/1
  Vq/1 -> Mux1/2, q/1
  Vd/1 -> Mux1/1, d/1
  Add1/1 -> Gain6/1
  Gain6/1 -> 0/1
  Mux1/1 -> Scope3/1

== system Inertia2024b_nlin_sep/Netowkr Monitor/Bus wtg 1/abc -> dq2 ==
  a : Inport
  b : Inport  Port=2
  c : Inport  Port=3
  Theta : Inport  Port=4
  Add1 : Sum  Inputs=+++
  Add10 : Sum  Inputs=+++
  Add11 : Sum  Inputs=+++
  Add4 : Sum  Inputs=+-
  Add8 : Sum
  Constant6 : Constant  Value=2/3*pi
  Constant7 : Constant  Value=2/3*pi
  Divide{6..11} (6 alike) : Product  Inputs=**
  Gain6 : Gain  Gain=1/3
  Mux1 : Mux  Inputs=2
  Scope3 : Scope
  Trigonometric Function : Trigonometry  Operator=cos
  Trigonometric Function1 : Trigonometry  Operator=cos
  Trigonometric Function2 : Trigonometry  Operator=cos
  Trigonometric Function3 : Trigonometry
  Trigonometric Function4 : Trigonometry
  Trigonometric Function5 : Trigonometry
  Vd : Gain  Gain=2/3
  Vq : Gain  Gain=2/3
  d : Outport  VectorParamsAs1DForOutWhenUnconnected=off
  q : Outport  Port=2  VectorParamsAs1DForOutWhenUnconnected=off
  0 : Outport  Port=3  VectorParamsAs1DForOutWhenUnconnected=off
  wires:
  Theta/1 -> Add4/1, Add8/1, Trigonometric Function/1, Trigonometric Function3/1  "wt"
  Constant6/1 -> Add4/2
  Add4/1 -> Trigonometric Function1/1, Trigonometric Function4/1
  Add8/1 -> Trigonometric Function2/1, Trigonometric Function5/1
  Trigonometric Function3/1 -> Divide7/2
  Trigonometric Function4/1 -> Divide9/2
  Trigonometric Function5/1 -> Divide11/2
  a/1 -> Divide6/1, Divide7/1, Add1/1
  Trigonometric Function/1 -> Divide6/2
  Trigonometric Function2/1 -> Divide10/2
  Trigonometric Function1/1 -> Divide8/2
  b/1 -> Divide8/1, Divide9/1, Add1/2
  c/1 -> Divide10/1, Divide11/1, Add1/3
  Constant7/1 -> Add8/2
  Divide6/1 -> Add10/1
  Divide8/1 -> Add10/2
  Divide10/1 -> Add10/3
  Divide7/1 -> Add11/1
  Divide9/1 -> Add11/2
  Divide11/1 -> Add11/3
  Add10/1 -> Vq/1
  Add11/1 -> Vd/1
  Vq/1 -> Mux1/2, q/1
  Vd/1 -> Mux1/1, d/1
  Add1/1 -> Gain6/1
  Gain6/1 -> 0/1
  Mux1/1 -> Scope3/1
